PROGRAM ModbusRTU_Slave
VAR
	ModbusRtuSlave:ModbusRtuSlave_Generic;

	(* The Input area is addressed with a 0 offset, i.e. address 0 as transferred in the telegram addresses the first element in the Input data area. *)
	Inputs  AT %IW0: ARRAY [1..100] OF WORD;	// 对应Modscan中的03,40001——40100
	(* The Output area is addressed with a 16#800 offset, i.e. address 16#800 as transferred in the telegram addresses the first element in the Output data area. *)
	Outputs AT %QW0: ARRAY [1..100] OF WORD;	// 对应Modscan中的03,42049——42149
	(* The Memory area is addressed with a 16#4000 offset, i.e. address 16#4000 as transferred in the telegram addresses the first word in the Memory data area. *)
	Memorys AT %MW0: ARRAY [1..100] OF WORD;	// 对应Modscan中的03,416385——416485
END_VAR

ModbusRtuSlave(
	UnitID:=1 , 
	AdrInputs:=ADR(Inputs) , 
	SizeInputBytes:=SIZEOF(Inputs) , 
	AdrOutputs:=ADR(Outputs) , 
	SizeOutputBytes:=SIZEOF(Outputs) , 
	AdrMemory:=ADR(Memorys) , 
	SizeMemoryBytes:=SIZEOF(Memorys) , 
	RxBuffer:=RxBuffer , 
	TxBuffer:=TxBuffer , 
	ErrorId=> );

END_PROGRAM
